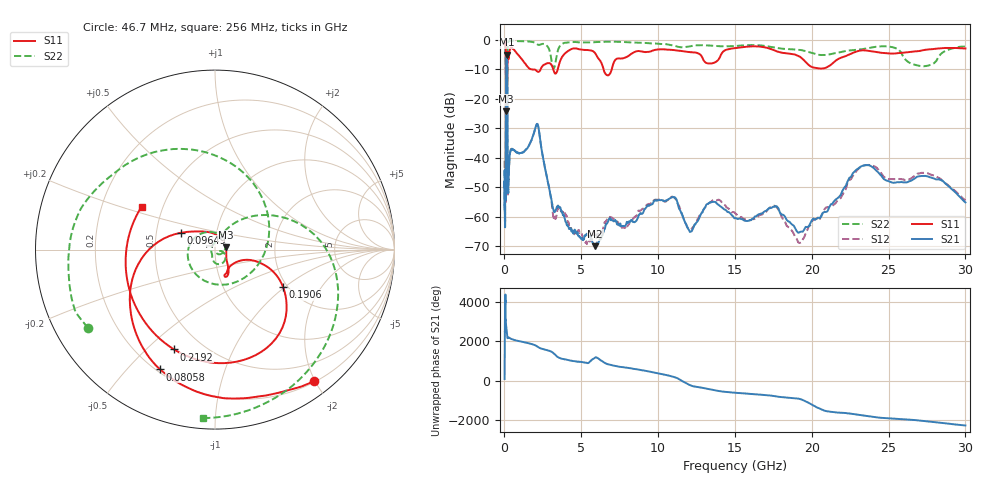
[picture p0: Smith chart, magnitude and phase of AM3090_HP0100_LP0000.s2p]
! Date/Time: Thu, Feb 28, 2019 1:57 PM
! Network Analyzer: Agilent Technologies E8364B Rev: A.07.50.67
! Sweep from 0.010 to 30.000 GHz, 1601 Points, Sweep Type: LOG
! Power Supply: 5.023 V, 0.002 A
# Hz S DB R 50
!freq MagS11 AngS11 MagS21 AngS21 MagS12 AngS12 MagS22 AngS22
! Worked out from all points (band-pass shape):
!   1601 points, 10 MHz to 30 GHz, reference 50 ohm
!   highest |S21| = -4.95 dB at 136.3 MHz (marker M1); lowest = -70.0 dB at 5.9 GHz (marker M2)
!   |S21| within 3 dB of the highest: 104 MHz to 174.7 MHz (70.73 MHz wide, 50.7 % of centre)
!   lowest |S11| = -24.2 dB at 103.5 MHz (marker M3), VSWR 1.13, Z = 56.4 + j1.46 ohm
!   |S11| at or under -10 dB: 1.952 GHz to 2.349 GHz (397 MHz wide, 18.5 % of centre); 3.182 GHz to 3.465 GHz (282.5 MHz wide, 8.5 % of centre); 6.454 GHz to 6.979 GHz (524.4 MHz wide, 7.81 % of centre)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
!   |S22| runs from -34.7 to -0.1 dB; largest |S21 - S12| = 0.012
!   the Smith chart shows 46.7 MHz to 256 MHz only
!   S11 on the Smith chart (normalised r, x): 46.7 MHz: 0.22, -1.98; 80.58 MHz: 0.21, -0.62; 96.49 MHz: 0.67, +0.13; 190.6 MHz: 1.89, -0.97; 219.2 MHz: 0.35, -0.61; 256 MHz: 0.38, +0.23
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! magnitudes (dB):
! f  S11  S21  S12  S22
! 10 MHz  -0.3  -45.9  -41.0  -0.5
! 38.04 MHz  -0.5  -59.9  -56.4  -1.3
! 46.7 MHz  -0.8  -51.3  -51.1  -1.6
! 80.58 MHz  -2.7  -46.6  -46.5  -5.6
! 96.49 MHz  -13.4  -14.0  -14.0  -15.0
! 103.5 MHz  -24.2  -8.2  -8.2  -17.9
! 136.3 MHz  -16.6  -5.0  -4.9  -32.9
! 144.7 MHz  -16.8  -5.0  -5.0  -23.3
! 170.7 MHz  -15.9  -7.0  -7.0  -33.4
! 190.6 MHz  -7.3  -20.8  -20.6  -9.2
! 205.4 MHz  -4.0  -46.2  -46.2  -2.7
! 219.2 MHz  -4.4  -51.3  -52.1  -1.4
! 256 MHz  -6.5  -50.7  -49.5  -0.5
! 550.5 MHz  -3.0  -37.2  -37.3  -0.2
! 2.084 GHz  -10.5  -28.8  -28.8  -1.2
! 3.236 GHz  -10.9  -58.1  -60.0  -9.4
! 5.9 GHz  -4.5  -70.0  -66.4  -0.7
! 7.926 GHz  -5.8  -62.5  -62.8  -0.7
! 10.76 GHz  -3.3  -53.8  -53.8  -1.6
! 19.22 GHz  -5.6  -65.3  -69.0  -3.4
! 23.48 GHz  -3.5  -42.5  -42.5  -2.9
! 30 GHz  -2.9  -55.2  -54.5  -2.2
